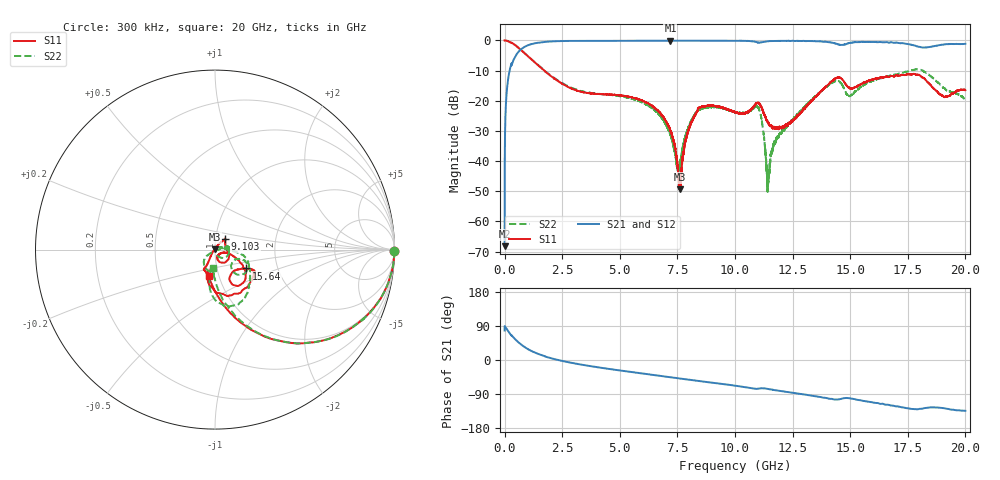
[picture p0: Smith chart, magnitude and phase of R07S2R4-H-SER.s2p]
!{R07S2R4}
!Johanson Technology Inc.
!www.johansontechnology.com
!Test Board Conditions:
!Substrate Type  RO4350B
!Substrate Thickness  10 mil
!Substrate Dk  3.66
!TL Type: GCPW
!TL Trace Width  21 mil
!TL Gap  20 mil
!Electrode orientation  Horizontal
!DUT TOPOLOGY	SERIES
!Mounting Pad LxW  16x21 mil
! Created Sat Feb  6 11:28:36 2021
# hz S ma R 50
! 2 Port Network Data from SP1.SP block
! freq  magS11  angS11  magS21  angS21  magS12  angS12  magS22  angS22
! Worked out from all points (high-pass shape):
!   20001 points, 300 kHz to 20 GHz, reference 50 ohm
!   highest |S21| = -0.03 dB at 7.195 GHz (marker M1); lowest = -68.2 dB at 300 kHz (marker M2)
!   |S21| within 3 dB of the highest: 698 MHz to end of sweep
!   lowest |S11| = -49.4 dB at 7.608 GHz (marker M3), VSWR 1.01, Z = 49.7 + j0.213 ohm
!   |S11| at or under -10 dB: 1.723251 GHz to 1.723613 GHz (362.1 kHz wide, 0.021 % of centre); 1.725 GHz to end of sweep
!   |S22| runs from -50.2 to 0.0 dB; largest |S21 - S12| = 0.013
!   S11 on the Smith chart (normalised r, x): 300 kHz: open; 9.103 GHz: 1.11, +0.13; 15.64 GHz: 1.38, -0.30; 20 GHz: 0.90, -0.27
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300000  0.9997 -0.4  0.0003878 77.7  0.0004879 91.0  1 -0.5
1.283e8  0.9807 -11.8  0.1935 78.5  0.1935 78.5  0.9793 -11.8
4.633e8  0.833 -35.0  0.5436 54.6  0.5436 54.5  0.835 -35.0
1.4533e9  0.3874 -74.2  0.9168 16.2  0.9163 16.2  0.3913 -72.5
3.3343e9  0.1407 -109.2  0.9866 -12.2  0.9863 -12.2  0.1447 -93.1
6.6673e9  0.06803 -119.2  0.9937 -41.2  0.9933 -41.2  0.06116 -141.5
7.1953e9  0.03163 -125.2  0.9962 -45.5  0.9942 -45.4  0.02718 -139.7
7.6083e9  0.003397 140.9  0.9939 -48.8  0.9939 -48.8  0.008669 -26.6
8.1613e9  0.04768 52.1  0.9919 -53.3  0.9918 -53.3  0.05061 12.1
9.1033e9  0.08185 46.1  0.9906 -60.7  0.9896 -60.7  0.07744 7.4
1.00003e10  0.06455 28.1  0.9897 -67.7  0.9884 -67.8  0.06479 9.6
1.10173e10  0.09226 -46.7  0.9251 -75.9  0.9253 -75.9  0.07559 -29.5
1.14433e10  0.04194 -72.0  0.9713 -76.6  0.971 -76.6  0.005087 31.5
1.18733e10  0.03439 -47.1  0.9831 -80.8  0.9833 -80.8  0.02527 35.2
1.33343e10  0.1006 -18.4  0.9745 -94.1  0.9742 -94.1  0.1047 -4.9
1.44063e10  0.2395 -45.8  0.8826 -104.2  0.8793 -104.0  0.2137 -31.5
1.49573e10  0.1645 -56.9  0.9066 -100.8  0.9051 -100.7  0.1206 -36.3
1.56413e10  0.2028 -31.1  0.9425 -108.6  0.9447 -108.5  0.1866 -22.2
1.66673e10  0.2474 -29.7  0.9203 -118.4  0.9255 -118.8  0.2552 -39.9
1.80713e10  0.2526 -79.5  0.7733 -128.7  0.7699 -128.7  0.3261 -78.1
1.90513e10  0.1174 -103.2  0.8549 -127.0  0.8546 -127.2  0.1643 -99.5
2e10  0.15 -102.7  0.88 -134.2  0.8759 -134.0  0.1036 -95.9
